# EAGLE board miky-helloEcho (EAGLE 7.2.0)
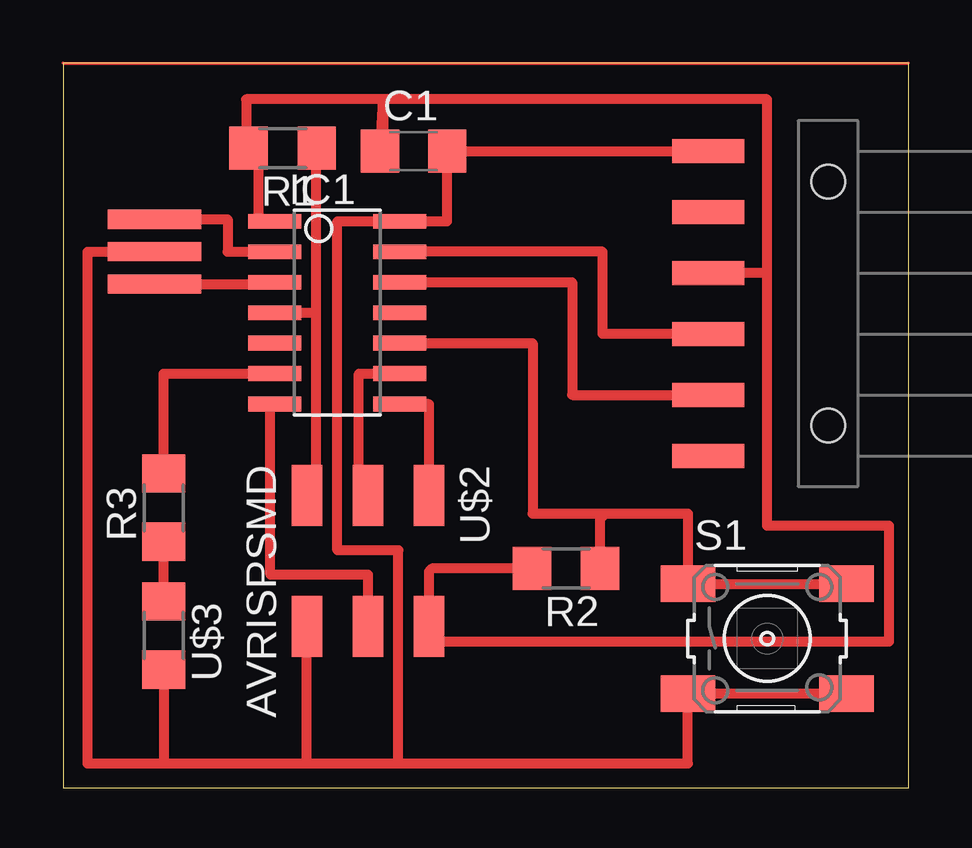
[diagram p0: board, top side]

Size 35.23 x 30.22 mm. Coordinates in mm from the lower left corner, seen from the top.
Outline: 0,0 35.23,0 35.23,30.22 0,30.22 0,0
Copper layers 1: Top 0.035mm
Design rules "ERP-1sided-10mil-16mill": minimum track width 10mil, minimum drill 24mil, track to track 16mil, track to pad 16mil, pad to pad 16mil, via to via 16mil, smd to smd 0mil, copper to edge 16mil, drill to drill 36mil, minimum pad ring 10mil, minimum via ring 8mil, stop-mask expansion 4mil, vias tented up to drill 0mil, thermal gap 10mil

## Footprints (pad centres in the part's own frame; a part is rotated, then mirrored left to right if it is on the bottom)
C1206 = smd 1.6 x 1.8: 1 -1.4,0; 2 1.4,0
SOIC14 = smd 0.61 x 2.21: 1 -3.81,-2.603; 2 -2.54,-2.603; 3 -1.27,-2.603; 4 0,-2.603; 5 1.27,-2.603; 6 2.54,-2.603; 7 3.81,-2.603; 8 3.81,2.603; 9 2.54,2.603; 10 1.27,2.603; 11 0,2.603; 12 -1.27,2.603; 13 -2.54,2.603; 14 -3.81,2.603
1X06-SMD = smd 1 x 3: 1 -6.35,5; 2 -3.81,5; 3 -1.27,5; 4 1.27,5; 5 3.81,5; 6 6.35,5 | hole 1.4: -5.08,0; 5.08,0
R1206 = smd 1.6 x 1.803: 1 -1.422,0; 2 1.422,0
1206 = smd 1.6 x 1.803: 1 -1.422,0; 2 1.422,0
6MM_SWITCH = smd 2.286 x 1.524: 1 -3.302,2.286; 2 3.302,2.286; 3 -3.302,-2.286; 4 3.302,-2.286
EFOBM = smd 0.8 x 3.9: 1 -1.35,0; 2 0,0; 3 1.35,0
2X03SMD = smd 2.54 x 1.27: 1 -2.54,2.54; 2 2.92,2.54; 3 -2.54,0; 4 2.92,0; 5 -2.54,-2.54; 6 2.92,-2.54

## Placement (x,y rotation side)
C1  1uf  [C1206]  14.61,26.54 0 top
IC1  ATTINY44-SSU  [SOIC14]  11.43,19.81 270 top
JP1  [1X06-SMD]  31.88,20.19 90 top
R1  10k  [R1206]  9.14,26.67 180 top
R2  [1206]  20.95,9.14 180 top
R3  2,6V  [R1206]  4.19,11.68 90 top
S1  [6MM_SWITCH]  29.34,6.22 0 top
U$1  RESONATOR  [EFOBM]  3.81,22.35 270 top
U$2  AVRISPSMD  [2X03SMD]  12.7,9.65 270 top
U$3  [1206]  4.19,6.35 270 top

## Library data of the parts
C1 = rcl
IC1 S1 U$1 U$2 = fab
JP1 = SparkFun
R1 R3 = resistor
R2 U$3 = ng

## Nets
BUTTON: IC1.10 R2.1 S1.1 S1.2
CTS: JP1.5
GND: C1.2 IC1.14 JP1.6 S1.3 S1.4 U$1.2 U$2.6 U$3.2
LED1: IC1.6 R3.2
MISO: IC1.8 U$2.1
MOSI: IC1.7 U$2.4
N$1: IC1.2 U$1.1
N$2: IC1.3 U$1.3
N$3: R3.1 U$3.1
RST: IC1.4 R1.1 U$2.5
RTS: JP1.1
RX: IC1.12 JP1.2
SCK: IC1.9 U$2.3
TX: IC1.13 JP1.3
VCC: C1.1 IC1.1 JP1.4 R1.2 R2.2 U$2.2

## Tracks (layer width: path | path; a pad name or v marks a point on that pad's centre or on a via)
BUTTON
  Top 0.406: IC1.10 19.56,18.54 19.56,11.43 22.61,11.43 | 22.61,11.43 26.04,11.43 S1.1 S1.2 | R2.1 22.38,11.2 22.61,11.43
GND
  Top 0.406: 13.97,1.02 13.97,9.91 11.43,9.91 11.43,23.62 IC1.14 16,23.62 16,26.67 C1.2 JP1.6 26.88,26.8 | 10.16,1.02 13.97,1.02 | U$1.2 1.02,22.35 1.02,1.02 4.19,1.02 | 4.19,1.02 10.16,1.02 | 10.16,1.02 U$2.6 | U$3.2 4.19,1.02 | 13.97,1.02 26.04,1.02 S1.3 S1.4
LED1
  Top 0.406: R3.2 4.19,17.27 IC1.6
MISO
  Top 0.406: IC1.8 15.24,16 U$2.1
MOSI
  Top 0.406: IC1.7 8.64,16 8.64,8.89 12.7,8.89 U$2.4
N$1
  Top 0.406: U$1.1 6.86,23.7 6.86,22.35 IC1.2
N$2
  Top 0.406: U$1.3 8.83,21 IC1.3
N$3
  Top 0.406: U$3.1 R3.1
RST
  Top 0.406: R1.1 10.54,26.67 10.54,19.81 | IC1.4 10.54,19.81 | U$2.5 10.54,12.19 10.54,19.81
RX
  Top 0.406: IC1.12 21.21,21.08 21.21,16.38 JP1.2
SCK
  Top 0.406: U$2.3 12.32,12.19 12.32,17.27 IC1.9
TX
  Top 0.406: JP1.3 22.48,18.92 22.48,22.35 IC1.13
VCC
  Top 0.254: 15.24,6.1 15.24,6.07
  Top 0.406: 29.34,21.46 JP1.4 | IC1.1 8.13,23.62 8.13,26.67 R1.2 7.62,26.67 7.62,28.7 13.33,28.7 C1.1 13.34,26.67 13.34,28.7 29.34,28.7 29.34,21.46 | R2.2 15.37,9.14 15.24,9.02 U$2.2 15.24,6.1 34.42,6.1 34.42,10.92 29.34,10.92 29.34,21.46
(copper drawn outside any net)
  shapes: Top area x1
